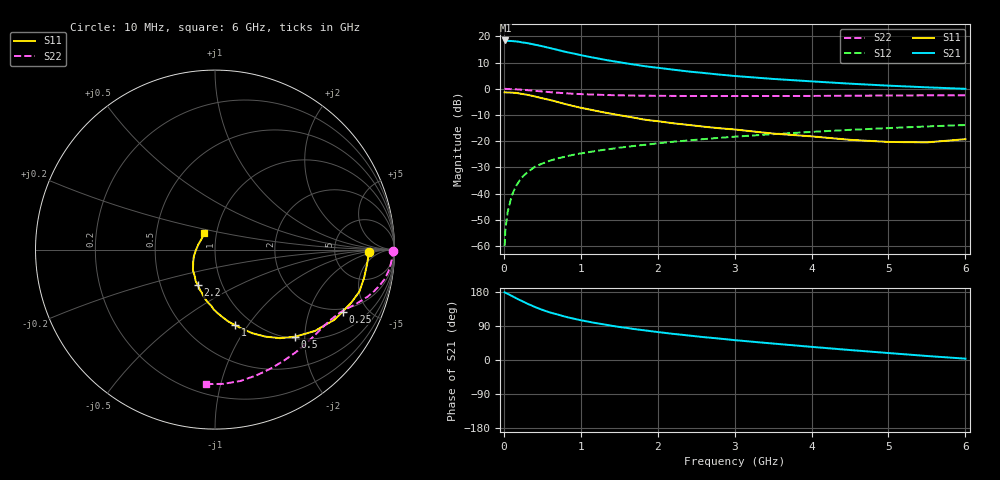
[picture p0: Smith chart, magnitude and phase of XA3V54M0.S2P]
! SIEMENS Discrete & RF Semiconductors
! BFY180
! Si NPN RF Bipolar Junction Transistor in MICRO-X
! VCE = 3.5 V  IC = 4 mA
! Common Emitter S-Parameters:  May  1997
# GHz  S  MA  R  50
!  f  S11  S21  S12  S22
! GHz  MAG  ANG  MAG  ANG  MAG  ANG  MAG  ANG
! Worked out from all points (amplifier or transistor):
!   36 points, 10 MHz to 6 GHz, reference 50 ohm
!   highest |S21| = 18.4 dB at 20 MHz (marker M1)
!   |S21| within 3 dB of that: start of sweep to 614.1 MHz
!   unconditionally stable (mu >= 1): 1.699 GHz to end of sweep
!   at 250 MHz: K = 0.24, MSG = 25.5 dB, |S12| = -33.3 dB
!   at 1.4 GHz: K = 0.92, MSG = 16.8 dB, |S12| = -22.9 dB
!   at 6 GHz: K = 1.08, MAG = 5.2 dB, |S12| = -13.8 dB
!   S11 on the Smith chart (normalised r, x): 10 MHz: 13, -1; 250 MHz: 1.85, -3.41; 500 MHz: 1.04, -1.79; 1 GHz: 0.84, -0.87; 2.2 GHz: 0.77, -0.32; 6 GHz: 0.87, +0.16
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0.01  0.8594 -0.9  8.249 178.5  0.001 89.7  0.9907 -0.3
0.02  0.8561 -2.1  8.349 177.4  0.0021 87.3  0.9999 -0.9
0.05  0.8513 -5.4  8.187 174.7  0.0045 86.4  0.9902 -2.0
0.1  0.8453 -10.8  8.158 169.4  0.0089 82.4  0.9837 -4.3
0.2  0.8158 -21.0  7.863 159.0  0.0174 78.0  0.9683 -8.2
0.25  0.7913 -25.9  7.616 154.2  0.0216 75.2  0.9574 -10.1
0.3  0.7712 -30.5  7.453 149.2  0.0251 73.4  0.9436 -11.7
0.4  0.7174 -39.2  6.961 140.3  0.0324 68.6  0.917 -14.6
0.5  0.6593 -47.4  6.475 132.4  0.0377 65.1  0.8892 -17.2
0.6  0.6122 -53.7  5.979 125.4  0.0426 62.5  0.8635 -19.2
0.8  0.5114 -65.8  5.066 114.2  0.051 58.4  0.8226 -22.6
1  0.4355 -75.2  4.392 104.9  0.0586 55.6  0.7922 -25.4
1.1  0.4068 -79.6  4.091 101.1  0.0618 54.8  0.7812 -26.6
1.3  0.3549 -87.5  3.602 94.0  0.0687 53.3  0.764 -29.3
1.5  0.3141 -93.8  3.217 87.2  0.0754 52.2  0.7515 -31.9
1.7  0.2804 -101.2  2.892 81.5  0.0816 51.4  0.7421 -34.5
2.2  0.2203 -115.6  2.318 69.0  0.0978 48.3  0.732 -41.2
2.8  0.1773 -131.6  1.868 56.6  0.1162 45.1  0.7279 -49.1
3.5  0.1402 -150.1  1.543 43.4  0.1366 40.3  0.7283 -58.5
4.5  0.1065 -178.4  1.253 26.3  0.165 32.9  0.7381 -72.0
5.5  0.0952 142.7  1.067 10.6  0.1916 25.2  0.7495 -86.5
6  0.1096 123.4  0.999 3.5  0.2039 21.0  0.7509 -93.7
